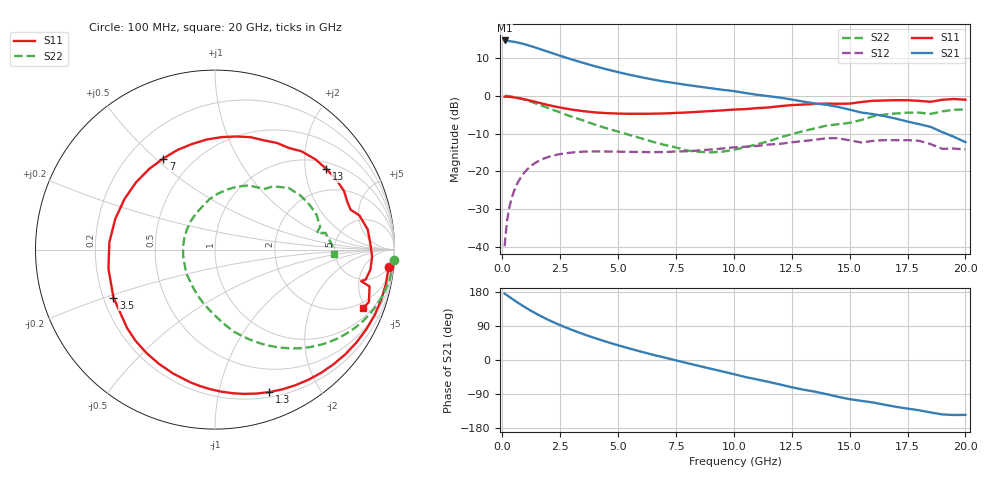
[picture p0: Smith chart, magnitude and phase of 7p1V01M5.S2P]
! Infineon Technologies  Discrete & RF Semiconductors
! bfp620
! VCE =  1.0 V,  IC =  1.5 mA
! Common Emitter S-Parameters:  Sep 2002
# GHz  S  MA  R  50
!  f  S11  S21  S12  S22
! GHz  MAG  ANG  MAG  ANG  MAG  ANG  MAG  ANG
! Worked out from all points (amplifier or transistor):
!   59 points, 100 MHz to 20 GHz, reference 50 ohm
!   highest |S21| = 14.6 dB at 100 MHz (marker M1)
!   |S21| within 3 dB of that: start of sweep to 1.985 GHz
!   unconditionally stable (mu >= 1): 6.113 GHz to 15.82 GHz; 17.42 GHz to end of sweep
!   at 1 GHz: K = 0.14, MSG = 16.8 dB, |S12| = -19.9 dB
!   at 5.5 GHz: K = 0.90, MSG = 10.2 dB, |S12| = -14.8 dB
!   at 20 GHz: K = 1.64, MAG = -3.7 dB, |S12| = -14.2 dB
!   S11 on the Smith chart (normalised r, x): 100 MHz: 5, -18; 1.3 GHz: 0.25, -1.42; 3.5 GHz: 0.24, -0.21; 7 GHz: 0.34, +0.53; 13 GHz: 1.19, +2.59; 20 GHz: 1.54, -4.73
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0.1  0.9719 -5.8  5.381 175.2  0.0103 87.8  0.9984 -3.4
0.2  0.9714 -11.3  5.321 171.0  0.0217 83.6  0.9934 -6.8
0.3  0.9676 -16.9  5.269 166.8  0.0329 80.3  0.9857 -10.1
0.7  0.9314 -38.7  5.023 150.1  0.0743 66.7  0.9338 -22.6
1  0.8925 -54.3  4.761 138.6  0.1006 57.0  0.88 -31.1
1.3  0.8497 -69.1  4.466 127.8  0.1222 48.2  0.8205 -38.7
1.5  0.8205 -78.5  4.268 121.0  0.1339 42.8  0.7802 -43.3
1.8  0.7785 -91.8  3.98 111.6  0.1481 35.6  0.722 -49.6
2.4  0.7087 -116.3  3.453 94.5  0.1675 23.5  0.6175 -60.3
3  0.6564 -138.3  3.017 79.6  0.178 13.5  0.5293 -69.8
3.5  0.6257 -154.7  2.719 68.3  0.1829 6.5  0.4707 -76.9
4  0.6032 -169.8  2.457 57.8  0.1839 0.3  0.4157 -83.3
5  0.5815 162.9  2.053 38.8  0.1828 -8.5  0.3361 -95.6
6  0.578 139.6  1.76 21.9  0.1807 -15.0  0.2738 -110.5
7  0.5837 119.6  1.541 6.6  0.1805 -19.3  0.2244 -128.2
8.5  0.6151 94.3  1.322 -15.7  0.1895 -25.1  0.1813 -167.5
10.5  0.6671 65.8  1.088 -45.0  0.2123 -35.9  0.2087 130.1
13  0.7656 36.0  0.837 -78.2  0.2522 -51.8  0.3407 78.8
13.5  0.7799 30.3  0.792 -83.6  0.2619 -56.3  0.3705 70.9
15  0.7874 16.4  0.656 -103.3  0.2578 -76.5  0.4389 50.5
17  0.876 -2.5  0.499 -123.5  0.2586 -89.0  0.5837 25.1
20  0.8867 -21.7  0.244 -144.8  0.1947 -112.7  0.6608 -2.2
